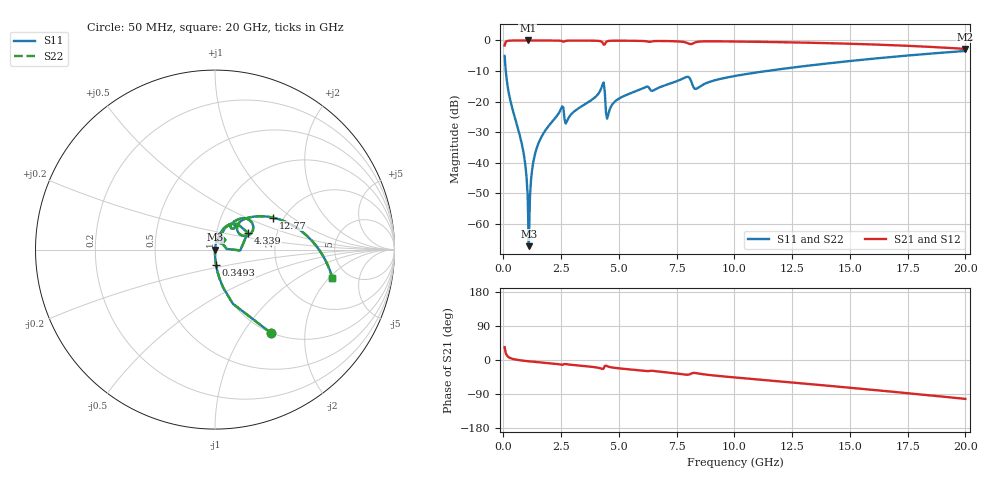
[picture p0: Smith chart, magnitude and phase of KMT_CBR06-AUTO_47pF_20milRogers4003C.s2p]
! Data measured by Modelithics Inc. support@modelithics.com 813-866-6335
! KEMET CBR06-AUTO 47pF, Pad Width= 0.851mm, Pad Length= 0.64mm, Pad Gap= 0.62mm, 20mil Rogers 4003C substrate Data, January 2022
# hz S ma R 50
! 2 Port Network Data from SP1.SP block
! freq  magS11  angS11  magS21  angS21  magS12  angS12  magS22  angS22
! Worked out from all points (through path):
!   401 points, 50 MHz to 20 GHz, reference 50 ohm
!   highest |S21| = 0.00 dB at 1.048 GHz (marker M1); lowest = -2.8 dB at 20 GHz (marker M2)
!   group delay of S21, straight-line fit = 14.5 ps
!   lowest |S11| = -67.3 dB at 1.097 GHz (marker M3), VSWR 1.00, Z = 50 - j0.00505 ohm
!   |S11| at or under -10 dB: 100.4 MHz to 11.39 GHz (11.29 GHz wide, 197 % of centre)
!   |S22| runs from -67.3 to -3.4 dB; largest |S21 - S12| = 0
!   S11 on the Smith chart (normalised r, x): 50 MHz: 1.00, -1.34; 349.2 MHz: 1.00, -0.17; 4.339 GHz: 1.41, +0.28; 12.77 GHz: 1.77, +0.73; 20 GHz: 3.77, -2.20
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5e7  0.5585 -56.2  0.8292 33.8  0.8292 33.8  0.5585 -56.2
3.4925e8  0.0866 -86.0  0.996 3.9  0.996 3.9  0.0866 -86.0
8.48e8  0.01617 -90.4  0.9995 -1.7  0.9995 -1.7  0.01617 -90.4
1.0475e9  0.00295 -84.9  0.9995 -3.1  0.9995 -3.1  0.00295 -84.9
1.097375e9  0.0004329 -6.7  0.9995 -3.4  0.9995 -3.4  0.0004329 -6.7
1.197125e9  0.005436 81.2  0.9995 -4.0  0.9995 -4.0  0.005436 81.2
1.247e9  0.008009 82.3  0.9995 -4.3  0.9995 -4.3  0.008009 82.3
1.34675e9  0.01294 82.9  0.9994 -4.9  0.9994 -4.9  0.01294 82.9
1.695875e9  0.02871 81.9  0.9989 -6.9  0.9989 -6.9  0.02871 81.9
2.493875e9  0.07624 69.6  0.9861 -12.1  0.9861 -12.1  0.07624 69.6
2.74325e9  0.04724 66.9  0.9891 -11.2  0.9891 -11.2  0.04724 66.9
3.391625e9  0.08424 73.5  0.9946 -15.4  0.9946 -15.4  0.08424 73.5
4.33925e9  0.2057 27.3  0.8548 -22.5  0.8548 -22.5  0.2057 27.3
4.53875e9  0.0621 55.3  0.9797 -17.5  0.9797 -17.5  0.0621 55.3
5.13725e9  0.1194 65.9  0.99 -22.8  0.99 -22.8  0.1194 65.9
6.73325e9  0.1694 57.3  0.9791 -30.6  0.9791 -30.6  0.1694 57.3
8.379125e9  0.1636 40.5  0.946 -35.0  0.946 -35.0  0.1636 40.5
1.0025e10  0.2626 43.1  0.9609 -46.1  0.9609 -46.1  0.2626 43.1
1.276812e10  0.3701 28.7  0.9255 -60.8  0.9255 -60.8  0.3701 28.7
1.336662e10  0.3939 25.4  0.9155 -64.1  0.9155 -64.1  0.3939 25.4
1.670825e10  0.5329 6.5  0.8403 -83.0  0.8403 -83.0  0.5329 6.5
2e10  0.6733 -13.7  0.7264 -102.7  0.7264 -102.7  0.6733 -13.7
